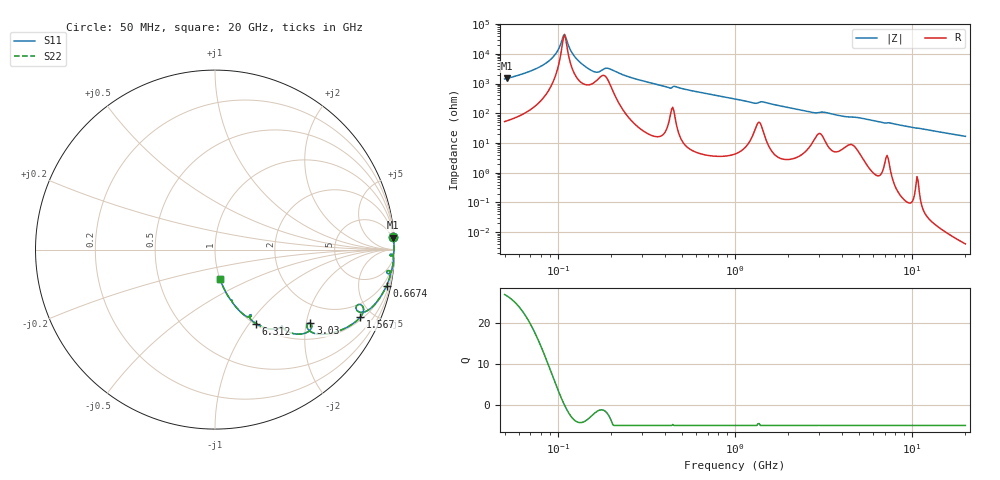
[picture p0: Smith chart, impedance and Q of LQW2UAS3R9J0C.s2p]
!Murata Part Number: LQW2UAS3R9J0C
!These Parameters are Measured in Series Mode Connection
!  o--[Z]--o
!Port1  Port2
!  o-------o
!Freq. Start=50[MHz] Stop=20[GHz], 401[Steps]
# Hz S RI R 50
!Freq.(Hz) S11(Real) S11(Imag) S21(Real) S21(Imag) S12(Real) S12(Imag) S22(Real) S22(Imag)
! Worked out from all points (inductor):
!   401 points, 50 MHz to 20 GHz, reference 50 ohm
!   read as one part in series: L = 3.51 uH near 51.52 MHz
!   highest Q = 26.7 at 51.52 MHz (marker M1), where L = 4.57 uH
!   self-resonance near 107.3 MHz
!   S11 on the Smith chart (normalised r, x): 50 MHz: 2, +28; 667.4 MHz: 1.08, -9.53; 1.567 GHz: 1.14, -4.23; 3.03 GHz: 1.41, -2.12; 6.312 GHz: 1.02, -1.08; 20 GHz: 1.00, -0.33
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5e7  0.9925 0.0699  0.00753 -0.0699  0.00753 -0.0699  0.9925 0.0699
5.152053e7  0.993 0.0668  0.00702 -0.0668  0.00702 -0.0668  0.993 0.0668
6.951576e7  0.9966 0.0385  0.00342 -0.0385  0.00342 -0.0385  0.9966 0.0385
8.573446e7  0.9978 0.0203  0.00223 -0.0203  0.00223 -0.0203  0.9978 0.0203
9.664883e7  0.998 0.0102  0.00202 -0.0102  0.00202 -0.0102  0.998 0.0102
1.057371e8  0.9979 0.00253  0.00213 -0.00253  0.00213 -0.00253  0.9979 0.00253
1.089527e8  0.9978 -6.47e-05  0.00223 6.47e-05  0.00223 6.47e-05  0.9978 -6.47e-05
1.209968e8  0.997 -0.00943  0.003 0.00943  0.003 0.00943  0.997 -0.00943
1.364002e8  0.9946 -0.021  0.00539 0.021  0.00539 0.021  0.9946 -0.021
1.608317e8  0.9812 -0.0349  0.0188 0.0349  0.0188 0.0349  0.9812 -0.0349
1.925012e8  0.9874 -0.0279  0.0126 0.0279  0.0126 0.0279  0.9874 -0.0279
2.520729e8  0.994 -0.0595  0.00605 0.0595  0.00605 0.0595  0.994 -0.0595
3.721004e8  0.9858 -0.1094  0.0142 0.1094  0.0142 0.1094  0.9858 -0.1094
6.673612e8  0.9563 -0.2002  0.0437 0.2002  0.0437 0.2002  0.9563 -0.2002
1e9  0.8985 -0.2951  0.1015 0.2951  0.1015 0.2951  0.8985 -0.2951
1.567309e9  0.8094 -0.3766  0.1906 0.3766  0.1906 0.3766  0.8094 -0.3766
2.728004e9  0.5291 -0.4546  0.4709 0.4546  0.4709 0.4546  0.5291 -0.4546
3.029571e9  0.532 -0.4107  0.468 0.4107  0.468 0.4107  0.532 -0.4107
3.572216e9  0.466 -0.4712  0.534 0.4712  0.534 0.4712  0.466 -0.4712
6.311513e9  0.2281 -0.4122  0.7719 0.4122  0.7719 0.4122  0.2281 -0.4122
7.442007e9  0.1934 -0.3758  0.8066 0.3758  0.8066 0.3758  0.1934 -0.3758
2e10  0.0273 -0.1628  0.9727 0.1628  0.9727 0.1628  0.0273 -0.1628
